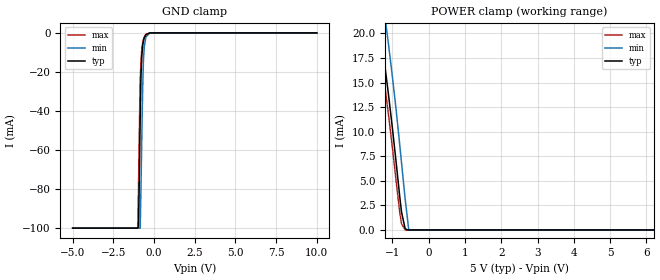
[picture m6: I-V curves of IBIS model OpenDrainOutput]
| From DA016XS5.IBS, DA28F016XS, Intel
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|*********************Open Drain Output Model*****************************
[Model]   OpenDrainOutput
Model_type   Open_drain
|   for RY/BY# pin 53
Vinl = 0.8V
Vinh = 2.0V
| Variable   typ   min   max
C_comp   9.61p   NA   11.6p
[Voltage Range]   5.0V   4.5V   5.5V
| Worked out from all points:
|   GND clamp passes 1 mA (typ) near -0.51 V on its own axis
|   POWER clamp passes 1 mA (typ) near -0.70 V on its own axis
[Pulldown]
| [Pullup] and [Pulldown] IV curves include only the current through
| the channels of output driver transistors when outputs are enabled
| with OE# = VIL.  Although the output driver transistors have np and
| pn diodes inherently created by CMOS IC fabrication between the
| drain and bulk of n-channel and p-channel CMOS transistors,
| the current through these junction diodes is not included in
| [Pullup] or [Pulldown].  Instead that drain/bulk diode current is
| included in the [POWER_clamp] or [GND_clamp] sections, which are
| not dependent on the state of OE# or output data value.  The RY/BY#
| Pulldown information is not provided for this device.  The table
| below is for the compatibility with some IBIS parsers.
|Voltage  I(typ)   I(min)   I(max)
-5V       0A         0A         0A
10V       0A         0A         0A
[GND_clamp]
| [POWER_clamp] and [GND_clamp] IV curves describe ESD protection
| circuits PLUS some np and pn diodes which exist between the
| drain and bulk of n-channel and p-channel CMOS transistors.
| These drain/bulk diodes are inherent in CMOS IC fabrication,
| and are visible on the node of the I/O pin at all times.
| Even the drain/bulk diodes of output driver [Pullup] and [Powerdown]
| transistors are included in [POWER_clamp] or [GND_clamp], because
| these diodes contribute to I/O pin current even when the
| chip outputs are tristated by OE# = VIH.
| For example, when V forced on the I/O pin is large, we are
| forward biasing the pn diode at the drain/bulk interface in the
| p-channel pullup transistor.  Similarly, when V forced on the
| I/O pin is sufficiently negative with respect to the substrate
| ground, we are forward biasing the np diode at the drain/bulk
| interface in the n-channel pulldown transistor.  The effects
| of these diodes are included in [POWER_clamp] or [GND_clamp].
|Voltage  I(typ)   I(min)   I(max)
-5V       -99.93mA   -99.94mA   -99.95mA
-1V       -99.93mA   -99.94mA   -99.95mA
-950mV    -98.62mA   -99.94mA   -76.39mA
-900mV    -71.02mA   -99.94mA   -47.61mA
-850mV    -43.05mA   -99.94mA   -24.04mA
-800mV    -21.14mA   -77.46mA   -13.76mA
-750mV    -11.8mA    -52.41mA   -7.934mA
-700mV    -6.593mA   -28.57mA   -5.011mA
-650mV    -3.982mA   -13.63mA   -3.323mA
-600mV    -2.493mA   -7.257mA   -2.154mA
-500mV    -885.4uA   -2.004mA   -725.7uA
10V       0A         0A         0A
[Pullup]
| (Voltages for [Pullup] and [POWER_clamp] are specified with
| negative respect to Vcc.  Reference the IBIS documentation
| for more information regarding Vtable = Vcc - Voutput.
| This method keeps -Vds constant for the values in all three
| columns across a line of the table.)
| [Pullup] and [Pulldown] IV curves include only the current through
| the channels of output driver transistors when outputs are enabled
| with OE# = VIL.  Although the output driver transistors have np and
| pn diodes inherently created by CMOS IC fabrication between the
| drain and bulk of n-channel and p-channel CMOS transistors,
| the current through these junction diodes is not included in
| [Pullup] or [Pulldown].  Instead that drain/bulk diode current is
| included in the [POWER_clamp] or [GND_clamp] sections, which are
| not dependent on the state of OE# or output data value.
|   Voltage  I(typ)   I(min)   I(max)
-5V       0A         0A         0A
10V       0A         0A         0A
[POWER_clamp]
| (Voltages for [Pullup] and [POWER_clamp] are specified with
| negative respect to Vcc.  Reference the IBIS documentation
| for more information regarding Vtable = Vcc - Voutput.
| This method keeps -Vds constant for the values in all three
| columns across a line of the table.
| [POWER_clamp] and [GND_clamp] IV curves describe ESD protection
| circuits PLUS some np and pn diodes which exist between the
| drain and bulk of n-channel and p-channel CMOS transistors.
| These drain/bulk diodes are inherent in CMOS IC fabrication,
| and are visible on the node of the I/O pin at all times.
| Even the drain/bulk diodes of output driver [Pullup] and [Powerdown]
| transistors are included in [POWER_clamp] or [GND_clamp], because
| these diodes contribute to I/O pin current even when the
| chip outputs are tristated by OE# = VIH.
| For example, when V forced on the I/O pin is large, we are
| forward biasing the pn diode at the drain/bulk interface in the
| p-channel pullup transistor.  Similarly, when V forced on the
| I/O pin is sufficiently negative with respect to the substrate
| ground, we are forward biasing the np diode at the drain/bulk
| interface in the n-channel pulldown transistor.  The effects
| of these diodes are included in [POWER_clamp] or [GND_clamp].
|Voltage  I(typ)   I(min)   I(max)
-5V       99.99mA    99.98mA    99.97mA
-1.5V     24.62mA    29.42mA    22.52mA
-1.4V     22.02mA    26.9mA     19.92mA
-1.3V     19.3mA     24.26mA    17.21mA
-1.2V     16.48mA    21.53mA    14.42mA
-1.1V     13.51mA    18.65mA    11.47mA
-900mV    6.963mA    12.29mA    5.052mA
-800mV    3.451mA    8.722mA    1.823mA
-750mV    1.84mA     6.854mA    639.6uA
-650mV    142.3uA    3.165mA    16.58uA
-550mV    0A         0A         0A
10V       0A         0A         0A
[Ramp]
| The RY/BY# Ramp information is not provided for this device.  The table
| below is for the compatibility with some IBIS parsers.
| Variable   typ   min   max
 dV/dt_r   0V/0ns   0V/0ns   0V/0ns
 dV/dt_f   0V/0ns   0V/0ns   0V/0ns
